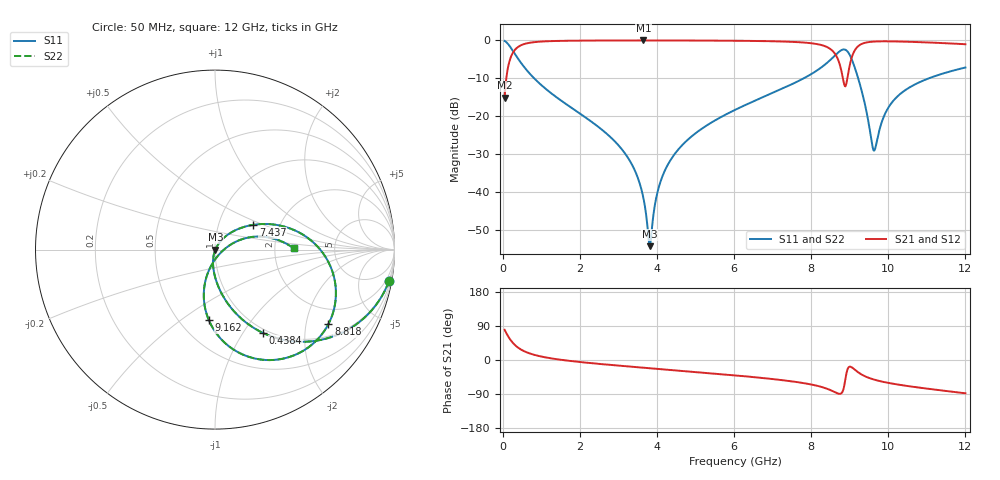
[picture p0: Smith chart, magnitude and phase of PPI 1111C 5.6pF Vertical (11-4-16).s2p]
# GHz S MA R 50
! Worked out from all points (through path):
!   1601 points, 50 MHz to 12 GHz, reference 50 ohm
!   highest |S21| = -0.02 dB at 3.65 GHz (marker M1); lowest = -15.2 dB at 50 MHz (marker M2)
!   group delay of S21, straight-line fit = 23.9 ps
!   lowest |S11| = -54.3 dB at 3.814 GHz (marker M3), VSWR 1.00, Z = 50.2 - j0.0743 ohm
!   |S11| at or under -10 dB: 814.8 MHz to 7.811 GHz (6.996 GHz wide, 162 % of centre); 9.219 GHz to 11.06 GHz (1.838 GHz wide, 18.1 % of centre)
!   |S22| runs from -54.3 to -0.1 dB; largest |S21 - S12| = 0
!   S11 on the Smith chart (normalised r, x): 50 MHz: 1, -11; 438.4 MHz: 0.95, -1.24; 7.437 GHz: 1.47, +0.43; 8.818 GHz: 1.39, -2.70; 9.162 GHz: 0.69, -0.64; 12 GHz: 2.56, +0.05
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0.05  0.9846 -10.4  0.1748 79.6  0.1748 79.6  0.9846 -10.4
0.199375  0.8155 -36.5  0.5784 53.5  0.5784 53.5  0.8155 -36.5
0.438375  0.5365 -60.0  0.8433 29.9  0.8433 29.9  0.5365 -60.0
0.9313125  0.277 -79.1  0.9599 10.7  0.9599 10.7  0.277 -79.1
2.044156  0.1045 -95.0  0.9931 -5.7  0.9931 -5.7  0.1045 -95.0
3.157  0.03296 -103.2  0.9976 -16.1  0.9976 -16.1  0.03296 -103.2
3.649938  0.008264 -97.3  0.9979 -20.3  0.9979 -20.3  0.008264 -97.3
3.81425  0.001917 -22.7  0.9979 -21.7  0.9979 -21.7  0.001917 -22.7
4.038312  0.01102 56.0  0.9977 -23.5  0.9977 -23.5  0.01102 56.0
4.665687  0.04188 58.2  0.9966 -28.7  0.9966 -28.7  0.04188 58.2
6.025  0.1208 48.0  0.9892 -40.5  0.9892 -40.5  0.1208 48.0
7.436594  0.2545 32.9  0.9596 -55.5  0.9596 -55.5  0.2545 32.9
8.019156  0.3633 22.4  0.9149 -65.0  0.9149 -65.0  0.3633 22.4
8.519562  0.5655 2.4  0.7547 -80.3  0.7547 -80.3  0.5655 2.4
8.818312  0.7559 -33.3  0.3255 -82.5  0.3255 -82.5  0.7559 -33.3
8.893  0.7498 -48.1  0.2498 -47.3  0.2498 -47.3  0.7498 -48.1
8.975156  0.677 -65.3  0.404 -19.0  0.404 -19.0  0.677 -65.3
9.161875  0.3926 -95.1  0.7795 -28.0  0.7795 -28.0  0.3926 -95.1
9.624937  0.03508 -46.7  0.9645 -51.5  0.9645 -51.5  0.03508 -46.7
10.01331  0.1322 21.0  0.9716 -60.6  0.9716 -60.6  0.1322 21.0
10.69297  0.2623 16.1  0.9529 -71.4  0.9529 -71.4  0.2623 16.1
12  0.4384 1.0  0.8897 -87.8  0.8897 -87.8  0.4384 1.0
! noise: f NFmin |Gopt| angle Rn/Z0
0.05  0.0004399  0.8969  2.426  0.0009315
1.372  0.003869  0.6829  8.673  0.002351
2.701  0.006366  0.6352  15.81  0.003227
4.031  0.00875  0.6159  22.79  0.004082
5.36  0.01145  0.6189  29.53  0.005256
6.682  0.0158  0.6586  36.09  0.008027
8.012  0.03423  0.8021  43.1  0.03111
9.341  0.0771  0.8963  50.09  0.1333
10.67  0.03174  0.7466  55.42  0.01986
12  0.02917  0.7115  60.17  0.01506
